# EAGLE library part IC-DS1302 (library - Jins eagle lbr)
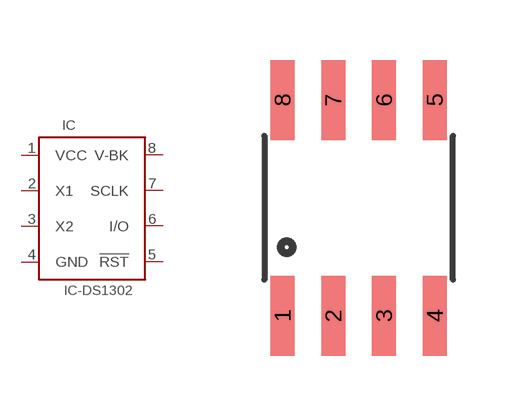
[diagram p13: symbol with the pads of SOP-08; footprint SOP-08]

Designator prefix IC

## IC-DS1302-RTC  [SOP-08]
1  VCC
2  X1
3  X2
4  GND
5  !RST
6  I/O
7  SCLK
8  V-BK

## Footprint SOP-08 (pad centres in mm)
smd 0.6 x 2: 1 -1.905,-2.7; 2 -0.635,-2.7; 3 0.635,-2.7; 4 1.905,-2.7; 5 1.905,2.7; 6 0.635,2.7; 7 -0.635,2.7; 8 -1.905,2.7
